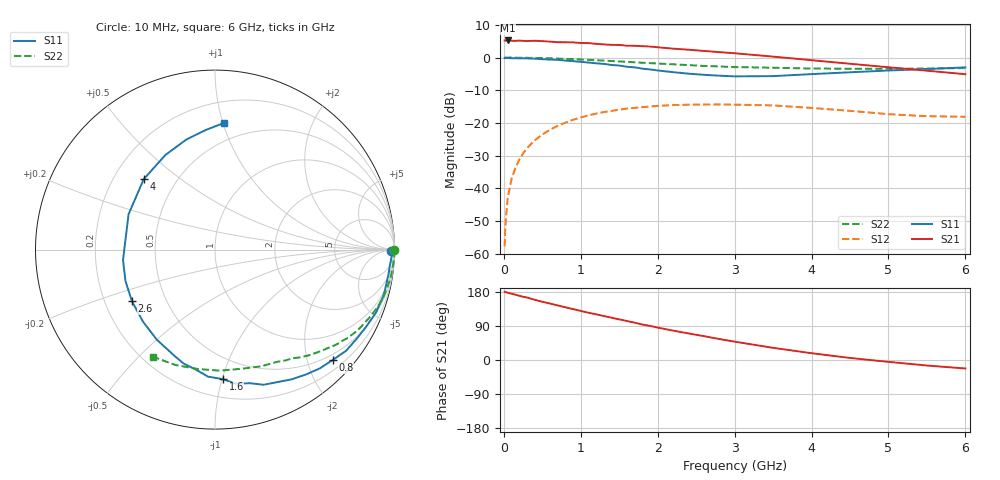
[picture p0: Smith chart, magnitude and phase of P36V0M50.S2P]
! SIEMENS Small Signal Semiconductors
! BFP181
! Si NPN RF Bipolar Junction Transistor in SOT143
! VCE = 6 V  IC = 0.5 mA
! Common Emitter S-Parameters:  March  1996
# GHz  S  MA  R  50
!  f  S11  S21  S12  S22
! GHz  MAG  ANG  MAG  ANG  MAG  ANG  MAG  ANG
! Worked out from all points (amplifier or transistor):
!   36 points, 10 MHz to 6 GHz, reference 50 ohm
!   highest |S21| = 5.2 dB at 50 MHz (marker M1)
!   |S21| within 3 dB of that: start of sweep to 2.491 GHz
!   unconditionally stable (mu >= 1): 3.827 GHz to end of sweep
!   at 250 MHz: K = 0.08, MSG = 17.2 dB, |S12| = -29.3 dB
!   at 1.4 GHz: K = 0.42, MSG = 10.1 dB, |S12| = -16.3 dB
!   at 6 GHz: K = 1.44, MAG = 2.6 dB, |S12| = -18.1 dB
!   S11 on the Smith chart (normalised r, x): 10 MHz: 80, -43; 800 MHz: 0.39, -2.47; 1.6 GHz: 0.33, -1.01; 2.6 GHz: 0.32, -0.26; 4 GHz: 0.33, +0.37; 6 GHz: 0.36, +1.01
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0.01  0.9808 -0.6  1.825 179.8  0.0013 70.6  0.9987 -0.2
0.02  0.9886 -1.1  1.822 179.5  0.0027 86.5  0.9986 -0.6
0.05  0.9847 -2.4  1.828 177.5  0.0071 91.0  0.9985 -1.3
0.1  0.9776 -5.5  1.812 174.9  0.0139 84.5  0.9999 -2.6
0.15  0.9764 -8.2  1.8 172.4  0.0204 83.5  0.9963 -4.0
0.2  0.9737 -10.9  1.823 169.6  0.0273 81.7  0.9951 -5.2
0.3  0.9713 -16.1  1.791 165.0  0.0409 78.9  0.9925 -7.9
0.4  0.9627 -21.5  1.809 159.0  0.054 75.0  0.9876 -10.5
0.5  0.9446 -27.3  1.785 153.7  0.0664 70.7  0.9806 -13.0
0.8  0.8991 -43.2  1.717 139.2  0.1009 59.6  0.9557 -20.4
1.1  0.8393 -59.5  1.667 124.7  0.1307 48.9  0.9225 -27.4
1.5  0.7555 -81.4  1.56 107.2  0.1594 36.3  0.8724 -35.7
1.6  0.7231 -86.5  1.52 102.9  0.1657 33.6  0.8624 -37.5
1.9  0.6584 -105.4  1.475 89.9  0.1781 25.0  0.8214 -43.1
2.2  0.5978 -122.8  1.369 77.5  0.1875 17.6  0.7896 -48.1
2.6  0.5449 -148.2  1.264 63.0  0.1912 8.8  0.7444 -54.4
3  0.5156 -173.6  1.164 48.4  0.1904 0.3  0.7158 -60.7
3.5  0.5202 157.8  1.035 32.1  0.1852 -8.0  0.6993 -68.5
4  0.5583 135.4  0.912 17.9  0.1696 -14.3  0.6799 -77.7
4.5  0.5954 117.6  0.804 5.4  0.1531 -18.6  0.6749 -87.8
5.5  0.668 94.5  0.63 -14.6  0.1268 -15.9  0.6796 -108.9
6  0.7074 86.0  0.557 -22.4  0.1241 -11.5  0.6897 -120.0
